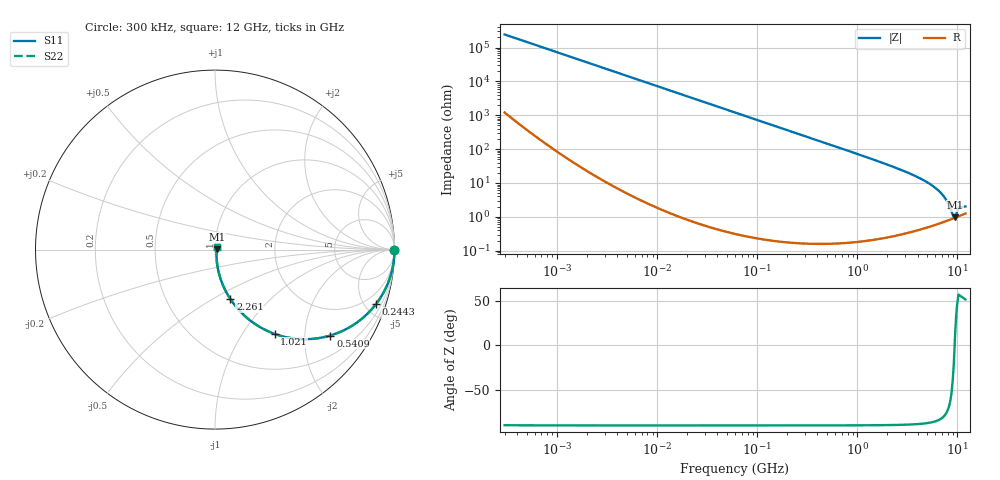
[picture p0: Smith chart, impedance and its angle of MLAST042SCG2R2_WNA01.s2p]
! MLAST042SCG2R2_WNA01  S-PARAMETER MODEL  ( General Type )
! Model Generated by TAIYO YUDEN Corporation (http://www.ty-top.com)
! Version 1.0
! TAIYO YUDEN Control No. 150820
! Copyright(c) 2015 TAIYO YUDEN CO.,LTD. All Rights Reserved.
! Product Description (link to TY-COMPAS)
! https://ds.yuden.co.jp/TYCOMPAS/or/detail?pn=MLAST042SCG2R2AWNA01&u=M
! Products Name : Multilayer Ceramic Capacitors
! Characteristics :
!  Capacitance : 2.2 pF , Rated Voltage : 25V , TCC : CG / C0G
!  Case Size : 0.4 x 0.2 / 0.016 x 0.008 [mm/inch] , Thickness : 0.2 / 0.008 [mm/inch]
!  (Conditions: Temperature = 25 degC , DC Bias Current/Voltage = 0A / 0V)
! External Node Assignments :
!  1  o---| |---o  2
! GND o---------o GND
! Frequency Range : 0.3MHz  -  12000MHz  [ 401 STEP ]
# MHz S RI R 50
! Freq[MHz].  S11 Real  S11 Imag  S21 Real  S21 Imag  S12 Real  S12 Imag  S22 Real  S22 Imag
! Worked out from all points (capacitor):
!   401 points, 300 kHz to 12 GHz, reference 50 ohm
!   read as one part in series: C = 2.19 pF near 316.3 kHz
!   lowest |Z| = 957 mohm at 9.454 GHz (marker M1)
!   series resonance near 9.369 GHz, so ESL is about 130 pH
!   S11 on the Smith chart (normalised r, x): 300 kHz: open; 244.3 MHz: 1.00, -5.95; 540.9 MHz: 1.00, -2.68; 1.021 GHz: 1.00, -1.41; 2.261 GHz: 1.01, -0.61; 12 GHz: 1.03, +0.03
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0.3  1 -0.000412  2.21e-06 0.000412  2.21e-06 0.000412  1 -0.000412
1.769972  1 -0.00243  7.57e-06 0.00243  7.57e-06 0.00243  1 -0.00243
10.44266  0.9998 -0.0143  0.000209 0.0143  0.000209 0.0143  0.9998 -0.0143
60  0.9932 -0.0819  0.00677 0.0819  0.00677 0.0819  0.9932 -0.0819
122.6847  0.9723 -0.1639  0.0277 0.1639  0.0277 0.1639  0.9723 -0.1639
244.3004  0.8985 -0.3017  0.1015 0.3017  0.1015 0.3017  0.8985 -0.3017
353.9943  0.8081 -0.3934  0.1919 0.3934  0.1919 0.3934  0.8081 -0.3934
540.8523  0.6426 -0.4786  0.3574 0.4786  0.3574 0.4786  0.6426 -0.4786
743.2595  0.4864 -0.499  0.5136 0.499  0.5136 0.499  0.4864 -0.499
1021.415  0.3319 -0.4696  0.6681 0.4696  0.6681 0.4696  0.3319 -0.4696
1441.349  0.1966 -0.3953  0.8034 0.3953  0.8034 0.3953  0.1966 -0.3953
2088.533  0.1007 -0.2972  0.8993 0.2972  0.8993 0.2972  0.1007 -0.2972
2261.293  0.0862 -0.2764  0.9138 0.2764  0.9138 0.2764  0.0862 -0.2764
4050.141  0.0247 -0.1421  0.9753 0.1421  0.9753 0.1421  0.0247 -0.1421
5868.704  0.0112 -0.0744  0.9888 0.0744  0.9888 0.0744  0.0112 -0.0744
7254.098  0.00858 -0.0399  0.9914 0.0399  0.9914 0.0399  0.00858 -0.0399
8064.993  0.00836 -0.0234  0.9916 0.0234  0.9916 0.0234  0.00836 -0.0234
8966.534  0.00883 -0.00716  0.9912 0.00716  0.9912 0.00716  0.00883 -0.00716
9207.246  0.00906 -0.00319  0.9909 0.00319  0.9909 0.00319  0.00906 -0.00319
9454.42  0.00933 0.00167  0.9907 -0.00167  0.9907 -0.00167  0.00933 0.00167
10511.28  0.0108 0.0155  0.9892 -0.0155  0.9892 -0.0155  0.0108 0.0155
12000  0.0126 0.0154  0.9874 -0.0154  0.9874 -0.0154  0.0126 0.0154
